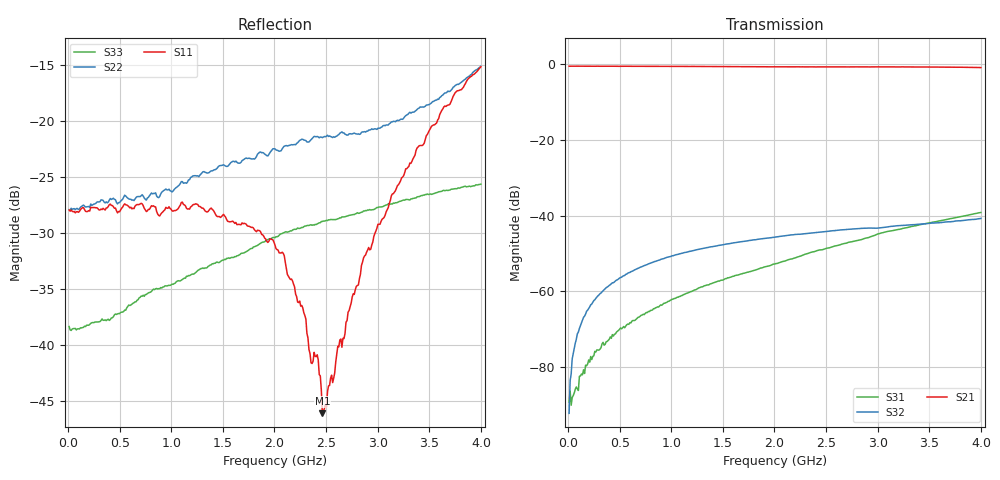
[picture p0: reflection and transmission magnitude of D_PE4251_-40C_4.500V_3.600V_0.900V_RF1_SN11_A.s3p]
! Device ID: PE4251_SoldCshunt_081809
! Dir: c:\Test Bench Repositories\Bench_Software_CVI_Version_8\trunk\PSC 4Port_VNA Bench\datalog\4250\TEST\PE4251_SoldCshunt_081809\-40C\4p500000\RF1
! Serial: 11
! Insertion: A
! Temp: -40C
! VDD: 4.500
! Control_Hi: 80.000
! Control_Lo: 20.000
! Logic State: RF1
! Port 1: RFC
! Port 2: RF1
! Port 3: RF2
! V1 = 0.90
! V2 = 3.60
! V3 = 0.90
! IDD: 5.568870e-05
! FILE NAME
! DATE 08/18/09  20:09
! CORRECTED  DATA
#  Hz  S  RI  R  50.00
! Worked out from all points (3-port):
!   401 points, 10 MHz to 4 GHz, reference 50 ohm
!   strongest paths, dB at 10 MHz, 1.008 GHz, 2.005 GHz, 3.002 GHz, 4 GHz:
!     S21: -0.5, -0.5, -0.6, -0.7, -0.9
!     S32: -92.2, -50.6, -45.7, -43.3, -40.7
!     S31: -89.2, -62.1, -52.7, -44.8, -39.2
!   lowest |S11| = -46.1 dB at 2.464 GHz (marker M1), VSWR 1.01, Z = 50.2 - j0.468 ohm
!   |S11| at or under -10 dB: start of sweep to end of sweep
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1e7  0.0401 0.000202  0.9453 -0.00334  5.51e-05 1.66e-05
     0.9453 -0.00545  0.0403 0.000234  -2.82e-05 6.49e-05
     -8.08e-07 -3.45e-05  1.17e-05 2.15e-05  0.0121 -0.000347
1.79575e8  0.0394 0.000773  0.9431 -0.0611  -1.07e-05 -9.73e-05
           0.9428 -0.0611  0.0414 0.000518  4.45e-05 0.000538
           -9.9e-06 -0.000103  3.58e-05 0.000544  0.0122 0.00158
4.888e8  0.0394 -0.00288  0.9286 -0.1628  -0.00016 -0.000258
         0.9288 -0.1617  0.0431 -0.00305  0.000144 0.00145
         -0.000158 -0.000261  0.000147 0.00145  0.0133 0.0039
1.0474e9  0.0378 -0.0133  0.8781 -0.3372  -0.000693 -0.000429
          0.8783 -0.3371  0.0489 -0.0124  0.000531 0.00299
          -0.000697 -0.000434  0.000549 0.003  0.0161 0.0103
2.005e9  0.026 -0.0102  0.7217 -0.5841  -0.00226 -0.000454
         0.7219 -0.5844  0.0663 -0.0354  0.00122 0.00506
         -0.00226 -0.000464  0.00121 0.00507  0.0184 0.0239
2.2843e9  0.0107 -0.00899  0.6664 -0.6439  -0.003 -0.000561
          0.6648 -0.6447  0.0645 -0.0512  0.00139 0.00558
          -0.00299 -0.000542  0.00137 0.00559  0.0169 0.0293
2.46385e9  0.00171 -0.00466  0.6295 -0.6794  -0.00351 -0.000491
           0.6281 -0.679  0.0615 -0.0578  0.00138 0.00592
           -0.00351 -0.000495  0.00138 0.00593  0.0155 0.0321
2.86285e9  -0.0179 -0.0168  0.5365 -0.7559  -0.00493 -0.000434
           0.5374 -0.7536  0.043 -0.0785  0.00152 0.00663
           -0.00493 -0.000425  0.0015 0.00664  0.0113 0.0381
3.14215e9  -0.0364 -0.0303  0.4643 -0.8003  -0.00633 -1.79e-05
           0.466 -0.799  0.0223 -0.0967  0.00118 0.00713
           -0.00634 -2.3e-05  0.00118 0.00714  0.00696 0.0421
4e9  -0.1568 -0.0772  0.1843 -0.89  -0.0108 0.00214
     0.1829 -0.8865  -0.1201 -0.1286  3.92e-05 0.00918
     -0.0108 0.00212  3.31e-05 0.0092  -0.0133 0.0506
